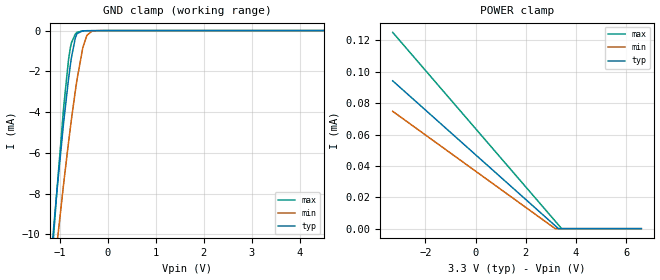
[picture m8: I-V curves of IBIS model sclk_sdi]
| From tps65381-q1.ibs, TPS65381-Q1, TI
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|   sclk_sdi Model
[Model]   sclk_sdi
Model_type   Input
Vinl = 0.99
Vinh = 2.31
|   typ   min   max
|   (nom PVT)   (fast PVT)   (slow PVT)
C_comp   8.028e-13   7.804e-13   8.085e-13
[Model spec]
|subparameter
Vinl   0.99   0.951   1.029
Vinh   2.31   2.219   2.401
| Where nom  PVT is Nominal Process, 3.3V, 27C
|   Fast PVT is Strong Process,  3.43V, -40C
|   Slow PVT is Weak Process,   3.17V, 150C
[Voltage Range]   3.3   3.17   3.43
|Junction Temperature
[Temperature Range]   27   150   -40
[Power Clamp Reference]   3.3   3.17   3.43
[GND Clamp Reference]   0   0   0
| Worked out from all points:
|   GND clamp passes 1 mA (typ) near -0.73 V on its own axis
[GND Clamp]
|   Voltage   I(typ)   I(min)   I(max)
-3.3V     -92.19mA   -76.99mA   -111.8mA
-1.228V   -12.38mA   -14.33mA   -13.37mA
-1.119V   -9.393mA   -11.8mA    -9.704mA
-1.059V   -7.83mA    -10.46mA   -7.797mA
-923mV    -4.541mA   -7.55mA    -3.821mA
-820.1mV  -2.393mA   -5.499mA   -1.441mA
-758.4mV  -1.316mA   -4.348mA   -597.9uA
-640.2mV  -146.5uA   -2.371mA   -83.47uA
-523.1mV  -12.05uA   -850.3uA   -12.58uA
-437.5mV  -6.579uA   -234.5uA   -8.269uA
-301.2mV  -4.303uA   -16.38uA   -5.598uA
6.6V      0A         0A         0A
[POWER Clamp]
|   Voltage   I(typ)   I(min)   I(max)
-3.3V     94.21uA    74.79uA    125.1uA
3.17V     1.856uA    0A         4.833uA
3.297V    47.11nA    0A         2.478uA
3.43V     0A         0A         0A
6.6V      0A         0A         0A
